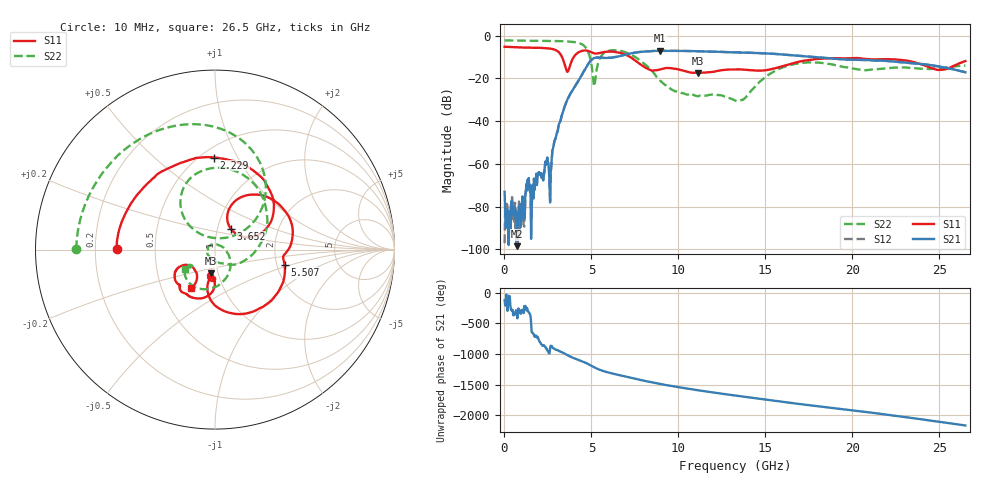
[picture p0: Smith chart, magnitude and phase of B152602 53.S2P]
!  2-Port S-parameters saved by WinCal
! VAR MeasName=S-Parameters (CALIBRATED_DATA) read from VNA (N5242A)
! VAR MeasDate=2016-1-5 16:33:36
! VAR NAME=B152602 53
! VAR FILENAME=B152602 53.S2P
! VAR DATE=2016-1-5 16:33:36
! VAR PHYS_PORTS=1,2
# Hz S DB R 50
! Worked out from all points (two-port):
!   801 points, 10 MHz to 26.5 GHz, reference 50 ohm
!   highest |S21| = -7.08 dB at 8.95 GHz (marker M1); lowest = -98.5 dB at 705.4 MHz (marker M2)
!   |S21| within 3 dB of the highest: 6.323 GHz to 17.85 GHz (11.53 GHz wide, 95.4 % of centre)
!   lowest |S11| = -17.4 dB at 11.1 GHz (marker M3), VSWR 1.31, Z = 46.1 - j12.4 ohm
!   |S11| at or under -10 dB: 3.311 GHz to 3.985 GHz (673.5 MHz wide, 18.5 % of centre); 7.236 GHz to end of sweep
!   |S22| runs from -30.6 to -2.2 dB; largest |S21 - S12| = 0.0032
!   S11 on the Smith chart (normalised r, x): 10 MHz: 0.29, +0.00; 2.229 GHz: 0.58, +0.80; 3.652 GHz: 1.16, +0.28; 5.507 GHz: 2.21, -0.44; 26.5 GHz: 0.70, -0.32
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1e7  -5.21 179.6  -73.06 -119.9  -97.04 -112.0  -2.24 179.8
7.053625e8  -5.44 152.5  -98.47 56.6  -90.45 -12.5  -2.27 169.1
2.228538e9  -5.80 90.7  -67.76 -143.7  -67.84 -153.1  -2.42 144.2
2.659e9  -6.09 68.8  -63.80 -143.0  -64.54 -146.2  -2.45 136.0
2.890788e9  -6.53 54.0  -48.89 160.2  -48.90 160.5  -2.49 131.2
3.652375e9  -16.69 53.3  -29.33 57.4  -29.34 57.4  -2.73 111.9
4.447075e9  -7.15 33.5  -18.38 -37.4  -18.38 -37.2  -3.99 77.2
4.811312e9  -7.17 9.6  -13.27 -83.1  -13.27 -82.9  -7.57 47.7
5.142438e9  -8.22 -3.9  -10.53 -133.8  -10.52 -133.6  -23.29 66.7
5.506675e9  -8.03 -12.3  -10.28 179.4  -10.29 179.5  -10.33 128.9
6.202038e9  -7.47 -42.4  -10.24 121.9  -10.24 122.0  -6.83 90.3
7.02985e9  -9.11 -80.4  -8.75 67.1  -8.72 67.2  -7.99 49.2
7.957e9  -14.16 -101.9  -7.49 7.4  -7.48 7.5  -12.59 1.3
8.851038e9  -16.02 -90.1  -7.09 -43.8  -7.06 -43.8  -20.21 -54.3
8.950375e9  -15.83 -89.6  -7.08 -49.2  -7.06 -49.3  -21.02 -60.9
1.110269e10  -17.42 -100.0  -7.29 -151.0  -7.27 -150.8  -28.33 177.5
1.3255e10  -15.82 -100.0  -7.81 122.1  -7.78 122.1  -30.35 107.6
1.56391e10  -15.10 -90.6  -8.59 31.3  -8.57 31.2  -16.05 -62.6
1.769208e10  -11.13 -103.7  -9.94 -42.7  -9.90 -42.6  -12.53 -121.5
2.209604e10  -10.99 -139.7  -11.93 163.8  -11.87 163.6  -15.13 -142.7
2.497682e10  -16.05 -140.1  -14.43 52.0  -14.40 52.0  -15.25 -143.8
2.65e10  -11.88 -122.1  -17.13 -7.9  -17.11 -8.2  -13.99 -147.7
